FUNCTION_BLOCK FB_Recipe_OtherHMI
VAR_INPUT
	bRunOnCeDevice				: BOOL	:= TRUE;	(*在CE系统运行*)
	sgFilePath					: STRING(255)	:= 'Data\Recipe\';	(*文件路径*)
	eFileType					: E_FileType	:= eFileType_XML;	(*文件类型, 只支持 eFileType_XML 和 eFileType_BIN 两种类型*)
(*配方和备份(用来比较配方参数是否修改的)的类型必须一致, 把两个变量的首地址和数据长度传到功能块*)
	pRecData					: PVOID;			(*配方首地址*)
	pBakData					: PVOID;			(*配方备份数据首地址, 数据类型必须和配方一样*)
	nRecSize					: UDINT;			(*配方的字节数*)
	tAutoSaveRec				: TIME	:= T#10S;	(*配方改变后, 延时保存*)

(*按钮, 下降沿触发!!!*)
	H_RecipeLoad				: BOOL;	(*读取设定配方号中的参数*)
	H_RecipeSave				: BOOL;	(*参数保存到当前配方号*)
	H_RecipeSaveAs				: BOOL;	(*参数保存到设定的配方号*)
(*设定配方号*)
	H_SetRecipeNum				: INT	:= 1;	(*设定配方号, 1~100*)
END_VAR
VAR_OUTPUT
(*当前配方号*)
	H_CurRecipeNum				: INT;
(*配方文件(和配方号对应的)名字*)
	H_CurRecName				: STRING(20);
(*状态*)
	H_RecipeInitialDone			: BOOL;	(*初始化完成*)
	H_RecipeDone				: BOOL;	(*读写完成*)
	H_RecipeBusy				: BOOL;	(*读写中*)
	H_RecipeError				: BOOL;	(*读写失败*)
	H_RecipeLoading				: BOOL;	(*配方读取中...*)
	H_RecipeSaving				: BOOL;	(*配方保存中...*)
	H_NewRecipeSaving			: BOOL;	(*配方另存中...*)
	H_CurDataAutoSaving			: BOOL;	(*自动保存中...*)
END_VAR
VAR_IN_OUT
	H_RecipeName				: ARRAY[0..MAX_RECIPE_FILES] OF STRING(MAX_FILE_NAME_STR);	(*0存放配方号, 1~MAX, 存放配方名字*)
END_VAR
VAR
	i: INT;
(*Last status*)
	s_sLastExecuteResult		: ST_LastExecutionResult_File;
(*FB*)
	s_fbRecipeManager			: FB_RecipeManager_2;
	s_sRecipeData				: ST_RecipeData_2;
	s_sRecipeCtrl				: ST_RecipeCtrl_2;	(*配方相关的命令和状态*)
(*上载配方动作, 上载完成后, 不判断当前参数是否有改变*)
	s_ftRecipeLoad				: F_TRIG;
	s_tonLoadRecipe				: TON;
(*参数改变, 延时触发写文件*)
	s_tonDataChange				: TON;
	s_bDataChange				: BOOL;
(*配方读写时间*)
	s_tActRecipeRead			: TIME;
	s_tActRecipeWrite			: TIME;
	s_tRecipeRead				: TIME;
	s_tRecipeWrite				: TIME;
	s_tonRecipeOperation		: TON;
	s_tonRecipeNotBusy			: TON;
END_VAR
(*第三方触摸屏*)
VAR
	tpRecipeLoad				: TP;
	tpRecipeSave				: TP;
	tpNewRecipeSave				: TP;
	fbFormatString				: FB_FormatString;
	bRecipeLoading				: BOOL;
	bRecipeSaving				: BOOL;
	bNewRecipeSaving			: BOOL;
	nLoadRecipeNum				: INT;		(*当前读取配方号*)
	fbWriteReadFile				: FB_WriteReadFileXML_ByAddr;	(*保存配方文件名和ID*)
	fbWriteReadFile_Bin			: FB_WriteReadFileBIN_2;
	tpInitialOk					: TP;
	bFileReadDone				: BOOL;
(*参数改变, 延时触发写文件*)
	s_sgRecipeName				: ARRAY[0..MAX_RECIPE_FILES] OF STRING(MAX_FILE_NAME_STR);	(*0存放配方号, 1~MAX, 存放配方名字*)
	s_tonRecipeNameChange		: TON;
	s_bRecipeNameChange			: BOOL;
	s_bRecipeNameChange1		: BOOL;
END_VAR

;
(*==================================================================
配置
==================================================================*)
	(*延时时间*)
	s_tonDataChange.PT					:= tAutoSaveRec;		(*参数修改后, 延时写入临时文件(作用是掉电保持)的时间*)
	s_tonRecipeNameChange.PT			:= tAutoSaveRec;
	s_tonLoadRecipe.PT					:= T#100MS;		(*上载配方时, 延时判断读取完成*)

	(*其他, 只针对TwinCAT PLC HMI, 第三方触摸屏的可以不设置*)
	s_sRecipeCtrl.i16DisplayFilesNum	:= 14;			(*Target Visualization中用到的'PH_RECIPE_FILE_NAME_DISPLAY'的数量, 如果是第三方HMI, 设置为0*)
	s_sRecipeCtrl.bRecipeNeedConfirm	:= TRUE;		(*上载, 保存, 删除是否需要确认. FALSE--不需要, TRUE--需要, 第三方触摸屏, 建议设置为FALSE*)	(*2020.10.10, 更改为FALSE*)
	s_sRecipeCtrl.bRecipeAutoRead		:= TRUE;		(*初始化时, 是否要从actRecipe中读取之前保存的参数*)
	s_sRecipeCtrl.bFileTypeDisplay		:= FALSE;		(*在'PH_RECIPE_FILE_NAME_DISPLAY'是否显示文件类型. FALSE--不显示, TRUE--显示*)
(*
	s_sRecipeCtrl.u16MaxTempFilesNum	:= 300;			(*保存300个临时文件*)
	s_sRecipeCtrl.u16KeepErrorFilesDay	:= 7;			(*错误文件保存7天*)
*)


(*==================================================================
变量地址是否有误
==================================================================*)
IF pRecData = 0 OR nRecSize <= 0 OR pBakData = 0 THEN
	H_RecipeError						:= TRUE;
	RETURN;
END_IF
(*变量的地址和长度*)
s_sRecipeData.stRecipeDataArr[1].pRecipeDataInfoADR			:= pRecData;
s_sRecipeData.stRecipeDataArr[1].u32RecipeDataInfoSIZEOF	:= nRecSize;
s_sRecipeData.stRecipeDataArr[1].sgRecipeDataInfoName		:= 'RecData';


(*==================================================================
第三方触摸屏
==================================================================*)
s_sRecipeCtrl.bRecipeNeedConfirm	:= FALSE;		(*上载, 保存, 删除是否需要确认. FALSE--不需要, TRUE--需要, 第三方触摸屏, 建议设置为FALSE*)	(*2020.10.10, 更改为FALSE*)
(*按钮, 在HMI设置保持2s后输出, 功能块中只接收下降沿, 所以用一个脉宽输出*)
tpRecipeLoad(IN := H_RecipeLoad, PT := T#50MS);
tpRecipeSave(IN := H_RecipeSave, PT := T#50MS);
tpNewRecipeSave(IN := H_RecipeSaveAs, PT := T#50MS);
(*配方号*)
H_SetRecipeNum := LIMIT(1, H_SetRecipeNum, MAX_RECIPE_FILES);
(*获取触摸屏按钮状态, 生成文件名, 并读写文件*)
IF NOT s_sRecipeCtrl.sStatus.bBusy THEN
	(*生成文件名*)
	IF tpRecipeLoad.Q THEN			(*读取设定配方号中的参数*)
		nLoadRecipeNum := H_SetRecipeNum;
		fbFormatString(
			sFormat:= 'Recipe_%.3d',
			arg1:= F_INT(H_SetRecipeNum),
			sOut=> s_sRecipeCtrl.sgFileNameLoad);
		bRecipeLoading := TRUE;
	ELSIF tpRecipeSave.Q THEN			(*参数保存到当前配方号*)
		fbFormatString(
			sFormat:= 'Recipe_%.3d',
			arg1:= F_INT(H_CurRecipeNum),
			sOut=> s_sRecipeCtrl.sgFileNameLoad);
		bRecipeSaving := TRUE;
	ELSIF tpNewRecipeSave.Q THEN		(*参数保存到设定的配方号*)
		fbFormatString(
			sFormat:= 'Recipe_%.3d',
			arg1:= F_INT(H_SetRecipeNum),
			sOut=> s_sRecipeCtrl.sgFileNameSave);
		bNewRecipeSaving := TRUE;
	END_IF
	(*命令*)
	s_sRecipeCtrl.sCmd.bRecipeLoad		:= tpRecipeLoad.Q;
	s_sRecipeCtrl.sCmd.bRecipeSave		:= tpRecipeSave.Q;
	s_sRecipeCtrl.sCmd.bRecipeSaveAs	:= tpNewRecipeSave.Q ;
END_IF

(*状态*)
H_RecipeInitialDone	:= s_sRecipeCtrl.sStatus.bInitialOk AND bFileReadDone;	(*初始化完成*)
H_RecipeLoading		:= s_sRecipeCtrl.sStatus.bBusy AND bRecipeLoading;		(*配方读取中...*)
H_RecipeSaving		:= s_sRecipeCtrl.sStatus.bBusy AND bRecipeSaving;			(*配方保存中...*)
H_NewRecipeSaving	:= s_sRecipeCtrl.sStatus.bBusy AND bNewRecipeSaving;		(*配方另存中...*)
H_CurDataAutoSaving	:= s_sRecipeCtrl.sStatus.bBusy							(*自动保存中...*)
						AND NOT (bRecipeLoading OR bRecipeSaving OR bNewRecipeSaving);
H_RecipeBusy		:= s_sRecipeCtrl.sStatus.bBusy							(*读写中*)
						AND (bRecipeLoading OR bRecipeSaving OR bNewRecipeSaving);
H_RecipeError		:= s_sRecipeCtrl.sStatus.bError;		(*读写失败*)
H_RecipeDone		:= s_sRecipeCtrl.sStatus.bDone;		(*读写完成*)
(*上一次触发的状态*)
MEMCPY(ADR(s_sLastExecuteResult), ADR(s_fbRecipeManager.s_sLastExecuteResult), SIZEOF(s_sLastExecuteResult));


(*显示当前使用的配方名*)
MEMSET(ADR(H_CurRecName), 0, SIZEOF(H_CurRecName));
MEMCPY(ADR(H_CurRecName), ADR(H_RecipeName[H_CurRecipeNum]), LEN(H_RecipeName[H_CurRecipeNum]));

(*读取成功后, 把当前配方号改为保存配方号*)
IF H_RecipeDone THEN
	bRecipeSaving := FALSE;
	IF bNewRecipeSaving THEN		(**)
		H_RecipeName[H_SetRecipeNum] := H_RecipeName[H_CurRecipeNum];		(*另存时, 复位当前配方名到新的配方号对应的配方名*)
		bNewRecipeSaving := FALSE;
	END_IF
	IF bRecipeLoading THEN
		bRecipeLoading := FALSE;
		H_CurRecipeNum := nLoadRecipeNum;
	END_IF
END_IF



(*==================================================================
判断参数是否变化, 变化后, 延时写入文件
==================================================================*)
s_tonRecipeNotBusy(IN := NOT s_sRecipeCtrl.sStatus.bBusy, PT := T#1S);
(*上载配方完成后, 把当前参数复制到临时参数中. 不写文件*)
s_ftRecipeLoad(CLK := s_sRecipeCtrl.sCmd.bRecipeLoad);
IF s_ftRecipeLoad.Q THEN
	s_tonLoadRecipe.IN := TRUE;
END_IF
s_tonLoadRecipe();
IF s_tonLoadRecipe.Q AND s_tonRecipeNotBusy.Q THEN
	s_tonLoadRecipe(IN := FALSE);
	s_tonDataChange(IN := FALSE);
END_IF

(*参数比较, 有变化时, 延时置位s_bDataChange, 将当前参数写到临时文件中*)
IF pRecData <> 0 AND nRecSize > 0 AND pBakData <> 0 THEN
	IF MEMCMP(pBakData, pRecData, nRecSize) <> 0 THEN
		s_tonDataChange(IN := FALSE);		(*重新计时*)
		s_tonDataChange(IN := s_sRecipeCtrl.sStatus.bInitialOk AND s_tonRecipeNotBusy.Q);	(*上载配方后, 只复制参数, 不写入临时文件*)
		MEMCPY(pBakData, pRecData, nRecSize);	(*比较不同, 重新定时, 并把数据复制到局部变量*)
	END_IF
END_IF

s_tonDataChange();
s_bDataChange := FALSE;
IF s_tonDataChange.Q AND s_tonRecipeNotBusy.Q THEN
	s_tonDataChange(IN := FALSE);
	s_bDataChange := TRUE;
END_IF

(*文件类型*)
IF eFileType = eFileType_BIN THEN
	s_fbRecipeManager.eFileType	:= eFileType_BIN;
ELSE
	s_fbRecipeManager.eFileType	:= eFileType_XML;
END_IF

(*==================================================================
调用配方程序, 根据实际情况修改文件夹路径: sgFolderName 和文件类型 eFileType
==================================================================*)
s_fbRecipeManager(
	sRecipeData				:= s_sRecipeData,		(*配方*)
	sgNetId					:= '',
	sgDeviceName			:= SEL(bRunOnCeDevice, 'C:\', '\Hard disk\'),		(*Device*)
	sgUsbDeviceName			:= SEL(bRunOnCeDevice, 'D:\', '\Hard disk2\'),		(*USB*)
	sgFolderName			:= sgFilePath,			(*文件夹, 支持多重, 写入时自动新建文件夹*)
	eFileType				:= ,					(*文件类型, 只支持 BIN 和 XML 两种类型*)
	bDataChange				:= s_bDataChange,		(*配方数据变更, 如果启用自动读取功能, 参数改变后, 会写到临时文件 actRecipe中, 掉电保持*)
	sRecipeCtrl				:= s_sRecipeCtrl);		(*和HMI的接口(按钮, 状态等)*)



(*记录读写时间*)
IF s_sRecipeCtrl.sStatus.bBusy THEN
	s_tonRecipeOperation(IN := TRUE, PT := T#1H);
	CASE s_fbRecipeManager.s_eOperateStep OF
		1..99:
			s_tActRecipeRead := s_tonRecipeOperation.ET;
		200..299:
			s_tActRecipeWrite := s_tonRecipeOperation.ET;
		300..399:
			s_tRecipeRead := s_tonRecipeOperation.ET;
		400..499:
			s_tRecipeWrite := s_tonRecipeOperation.ET;
	END_CASE
ELSE
	s_tonRecipeOperation(IN := FALSE);
END_IF


(*==================================================================
保存配方号和文件名
==================================================================*)
tpInitialOk(IN := s_sRecipeCtrl.sStatus.bInitialOk, PT := T#100MS);		(*读取配方参数后, 再读取文件名*)

IF bFileReadDone THEN
	H_RecipeName[0]		:= INT_TO_STRING(H_CurRecipeNum);
ELSE
	H_CurRecipeNum		:= STRING_TO_INT(H_RecipeName[0]);
END_IF

(*配方名比较, 有变化时, 延时置位s_bRecipeNameChange, 将当前配方名写到文件中*)
FOR i := 0 TO MAX_RECIPE_FILES BY 1 DO
	IF s_sgRecipeName[i] <> H_RecipeName[i] THEN
		s_sgRecipeName[i] := H_RecipeName[i];
		s_bRecipeNameChange1 := TRUE;
	END_IF
END_FOR
IF s_bRecipeNameChange1 THEN
	s_bRecipeNameChange1 := FALSE;
	s_tonRecipeNameChange(IN := FALSE);		(*重新计时*)
	s_tonRecipeNameChange(IN := s_sRecipeCtrl.sStatus.bInitialOk AND bFileReadDone);		(*上载配方后, 只复制参数, 不写入临时文件*)
END_IF

s_tonRecipeNameChange();

IF s_tonRecipeNameChange.Q AND s_tonRecipeNotBusy.Q THEN
	s_tonRecipeNameChange(IN := FALSE);
	s_bRecipeNameChange := TRUE;
END_IF


(*保存路径*)
	fbWriteReadFile.sgFilePath			:= F_CreatePath(s_fbRecipeManager.sgDeviceName, sgFilePath, '\name\', '');
	fbWriteReadFile_Bin.sgDeviceName	:= s_fbRecipeManager.sgDeviceName;
	fbWriteReadFile_Bin.sgFolderName	:= F_CreatePath(sgFilePath, '\name\', '', '');

CASE eFileType OF
	eFileType_BIN:
		fbWriteReadFile_Bin.sOption.bSameAddress_RW		:= TRUE;
		fbWriteReadFile_Bin.sOption.sBinHeader.bInused	:= FALSE;
		fbWriteReadFile_Bin(
			sgNetId:= '',
			sgDeviceName:= ,
			sgFolderName:= ,
			sgFileName:= 'RecipeName',
			bReadFile:= tpInitialOk.Q,
			pDestBuffer:= ADR(H_RecipeName),
			u32DestSize:= SIZEOF(H_RecipeName),
			bWriteFile:= s_bRecipeNameChange,
			pSrcBuffer:= ADR(H_RecipeName),
			u32SrcSize:= SIZEOF(H_RecipeName),
			sOption:= ,
			tTimeout:= T#5S,
			bBusy=> , 
			bDone=> , 
			bError=> ,
			u32ErrorID=> ,
			u32DestMaxRow=> , 
			u32DestMaxCol=> , 
			hFile=> );

		IF NOT fbWriteReadFile_Bin.bBusy AND s_sRecipeCtrl.sStatus.bInitialOk THEN
			bFileReadDone := TRUE;
			s_bRecipeNameChange := FALSE;
		END_IF
	ELSE
		fbWriteReadFile(
			bReadFile:= tpInitialOk.Q,
			bWriteFile:= s_bRecipeNameChange,
			sgFilePath:= ,
			sgFileName:= 'RecipeName.xml',
			pDataADR:= ADR(H_RecipeName),
			u32DataSIZEOF:= SIZEOF(H_RecipeName),
			sgVarName:= 'RecipeName',
			bBusy=> ,
			bError=> ,
			bDone=> );
		
		IF NOT fbWriteReadFile.bBusy AND s_sRecipeCtrl.sStatus.bInitialOk THEN
			bFileReadDone := TRUE;
			s_bRecipeNameChange := FALSE;
		END_IF
END_CASE

END_FUNCTION_BLOCK
